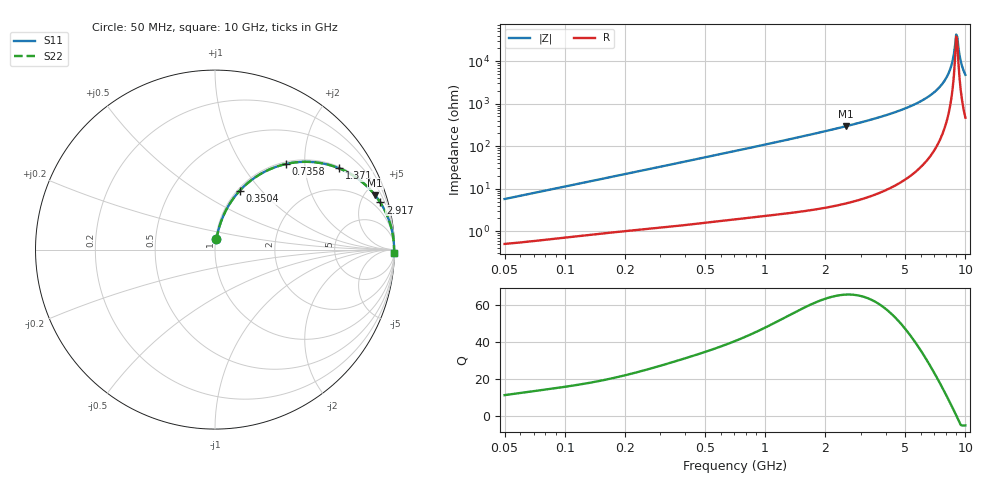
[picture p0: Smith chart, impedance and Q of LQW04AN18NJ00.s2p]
!Murata Part Number: LQW04AN18NJ00
!These Parameters are Measured in Series Mode Connection
!  o--[Z]--o
!Port1  Port2
!  o-------o
!Freq. Start=50[MHz] Stop=10[GHz], 401[Steps]
# Hz S RI R 50
!Freq.(Hz)	S 11(Real)	S 11(Imag)	S 21(Real)	S 21(Imag)	S 12(Real)	S 12(Imag)	S 22(Real)	S 22(Imag)
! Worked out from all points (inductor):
!   401 points, 50 MHz to 10 GHz, reference 50 ohm
!   read as one part in series: L = 18.1 nH near 51.34 MHz
!   highest Q = 65.5 at 2.522 GHz (marker M1), where L = 18.5 nH
!   self-resonance near 8.995 GHz
!   S11 on the Smith chart (normalised r, x): 50 MHz: 1.01, +0.11; 350.4 MHz: 1.03, +0.77; 735.8 MHz: 1.04, +1.60; 1.371 GHz: 1.05, +3.02; 2.917 GHz: 1.11, +6.98; 10 GHz: 10, -95
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5e7  0.0082 0.0563  0.9918 -0.0563  0.9918 -0.0563  0.0082 0.0563
1.214486e8  0.0255 0.1312  0.9745 -0.1312  0.9745 -0.1312  0.0255 0.1312
2.949953e8  0.1035 0.2866  0.8965 -0.2866  0.8965 -0.2866  0.1035 0.2866
3.504278e8  0.1366 0.3268  0.8634 -0.3268  0.8634 -0.3268  0.1366 0.3268
7.071068e8  0.3753 0.472  0.6247 -0.472  0.6247 -0.472  0.3753 0.472
7.357711e8  0.3936 0.4766  0.6064 -0.4766  0.6064 -0.4766  0.3936 0.4766
1.371241e9  0.6917 0.4528  0.3083 -0.4528  0.3083 -0.4528  0.6917 0.4528
1.717543e9  0.7816 0.4049  0.2184 -0.4049  0.2184 -0.4049  0.7816 0.4049
2.521925e9  0.8921 0.3027  0.1079 -0.3027  0.1079 -0.3027  0.8921 0.3027
2.917498e9  0.9207 0.2626  0.0793 -0.2626  0.0793 -0.2626  0.9207 0.2626
4.171863e9  0.9671 0.1698  0.0329 -0.1698  0.0329 -0.1698  0.9671 0.1698
5.88704e9  0.9893 0.0902  0.0107 -0.0902  0.0107 -0.0902  0.9893 0.0902
7.37379e9  0.996 0.0421  0.00403 -0.0421  0.00403 -0.0421  0.996 0.0421
7.878683e9  0.997 0.0284  0.00301 -0.0284  0.00301 -0.0284  0.997 0.0284
8.307378e9  0.9975 0.0174  0.00246 -0.0174  0.00246 -0.0174  0.9975 0.0174
8.530394e9  0.9977 0.012  0.00229 -0.012  0.00229 -0.012  0.9977 0.012
8.876195e9  0.9979 0.00377  0.00213 -0.00377  0.00213 -0.00377  0.9979 0.00377
8.994549e9  0.9979 0.00104  0.00211 -0.00104  0.00211 -0.00104  0.9979 0.00104
9.114482e9  0.9979 -0.00168  0.0021 0.00168  0.0021 0.00168  0.9979 -0.00168
9.236013e9  0.9979 -0.00441  0.00211 0.00441  0.00211 0.00441  0.9979 -0.00441
9.610418e9  0.9978 -0.0126  0.00223 0.0126  0.00223 0.0126  0.9978 -0.0126
1e10  0.9975 -0.0208  0.00249 0.0208  0.00249 0.0208  0.9975 -0.0208
